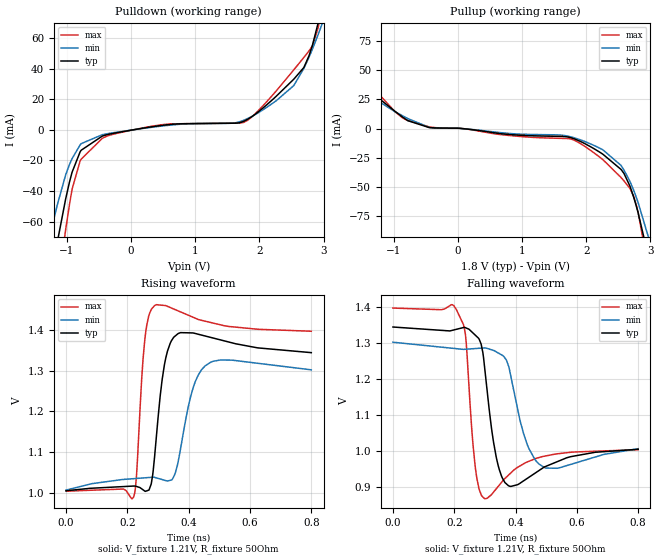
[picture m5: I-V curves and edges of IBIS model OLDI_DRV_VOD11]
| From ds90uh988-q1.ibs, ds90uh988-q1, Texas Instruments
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[Model]   OLDI_DRV_VOD11
Model_type   Output
Polarity   Non-Inverting
Vmeas = 0.55
Vref = 0.55
Cref = 0.02pF
Rref = 50
|   typ   min   max
C_comp   1.47pF   1.46pF   1.53pF
[Voltage Range]   1.8   1.71   1.89
[Temperature Range]   27   105   -40
[Pullup Reference]   1.8   1.71   1.89
[Pulldown Reference]   0   0   0
[Power Clamp Reference]   1.8   1.71   1.89
[GND Clamp Reference]   0   0   0
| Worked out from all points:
|   slope of the pulldown table from 0 to 0.27 V, typ, clamps not added: 145 ohm
|   slope of the pullup table from 0 to 0.27 V, typ, clamps not added: 172 ohm
|   falling waveform, V_fixture 1.21V, R_fixture 50Ohm: 20-80 % time 27.5ps typ, 46.5ps min, 18.3ps max; typ from 1.34 V to 1.01 V
|   rising waveform, V_fixture 1.21V, R_fixture 50Ohm: 20-80 % time 26.5ps typ, 46.3ps min, 17.2ps max; typ from 1.01 V to 1.34 V
[Pulldown]
|   Voltage   I(typ)   I(min)   I(max)
-1.8V     -234.3mA   -175.9mA   -318.4mA
-1.276V   -104.2mA   -72.33mA   -146.8mA
-1.147V   -73.58mA   -49.1mA    -105.1mA
-1.017V   -45.4mA    -29.6mA    -65.61mA
-914.4mV  -27.54mA   -18.69mA   -38.53mA
-774mV    -13.32mA   -9.011mA   -19.14mA
-217.8mV  -1.849mA   -1.531mA   -2.291mA
1.759V    5.596mA    6.287mA    4.892mA
2.536V    33.07mA    28.9mA     39.17mA
2.693V    40.68mA    40.1mA     47.3mA
2.92V     70.55mA    62.65mA    67.46mA
3.6V      244.2mA    148.5mA    433.9mA
[Pullup]
|   Voltage   I(typ)   I(min)   I(max)
-1.8V     86.8mA     75.94mA    75.74mA
-1.66V    54.98mA    57.84mA    59.43mA
-1.568V   43.54mA    46.92mA    51.4mA
-1.346V   31.12mA    27.42mA    36.68mA
-779.4mV  6.823mA    8.67mA     7.115mA
-444.6mV  893.6uA    994.1uA    1.478mA
1.975V    -12.76mA   -10.98mA   -15.1mA
2.542V    -34.95mA   -31.5mA    -41.84mA
2.687V    -50.3mA    -46.01mA   -51.84mA
2.812V    -72.88mA   -63.99mA   -72.66mA
3.006V    -118.6mA   -99.85mA   -131.8mA
3.6V      -270.5mA   -221.7mA   -333.2mA
[Ramp]
R_load = 50
|   typ   min   max
dV/dt_r   0.202985/2.64099e-11   0.176713/4.60817e-11   0.235067/1.71737e-11
dV/dt_f   0.202985/2.73437e-11   0.176713/4.56576e-11   0.235067/1.82676e-11
[Falling Waveform]
V_fixture = 1.21V
V_fixture_min = 1.21V
V_fixture_max = 1.21V
R_fixture = 50Ohm
C_fixture = 0F
|   Time   V(typ)   V(min)   V(max)
0s        1.344V     1.302V     1.396V
206.7ps   1.337V     1.284V     1.393V
235.4ps   1.342V     1.282V     1.329V
267.4ps   1.322V     1.284V     965.4mV
298ps     1.24V      1.286V     869.5mV
336.6ps   985.5mV    1.275V     895.8mV
376.8ps   904.7mV    1.237V     934mV
426.4ps   918.4mV    1.048V     965.5mV
476ps     946.5mV    965mV      982.7mV
800ps     1.006V     1.007V     1.005V
[Rising Waveform]
V_fixture = 1.21V
V_fixture_min = 1.21V
V_fixture_max = 1.21V
R_fixture = 50Ohm
C_fixture = 0F
|   Time   V(typ)   V(min)   V(max)
0s        1.006V     1.007V     1.005V
220.1ps   1.017V     1.035V     990.1mV
229.5ps   1.016V     1.036V     1.04V
256.2ps   1.005V     1.037V     1.371V
289.2ps   1.093V     1.038V     1.46V
323ps     1.323V     1.031V     1.459V
365.3ps   1.39V      1.076V     1.446V
406.5ps   1.392V     1.237V     1.433V
454ps     1.385V     1.312V     1.421V
800ps     1.344V     1.302V     1.396V
